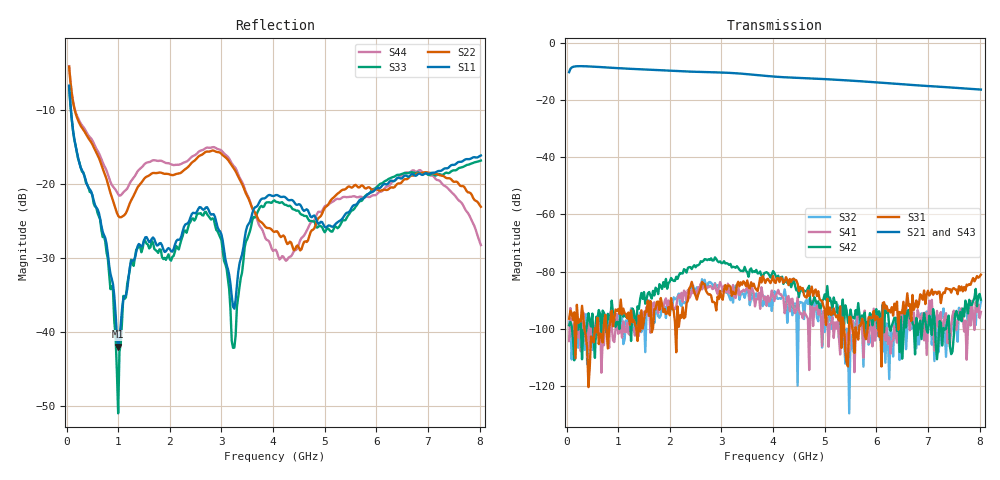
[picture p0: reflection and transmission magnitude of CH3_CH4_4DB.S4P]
!Agilent Technologies,E5071C,MY46316741,A.11.02
!Date: Thu May 28 15:03:34 2026
!Data & Calibration Information:
!1:CH3 INPUT 2:CH3 OUTPUT 3:CH4 INPUT 4:CH4 OUTPUT
!Freq	S11:SOLT4(ON)	S12:SOLT4(ON)	S13:SOLT4(ON)	S14:SOLT4(ON)
!	S21:SOLT4(ON)	S22:SOLT4(ON)	S23:SOLT4(ON)	S24:SOLT4(ON)
!	S31:SOLT4(ON)	S32:SOLT4(ON)	S33:SOLT4(ON)	S34:SOLT4(ON)
!	S41:SOLT4(ON)	S42:SOLT4(ON)	S43:SOLT4(ON)	S44:SOLT4(ON)
!PortZ  Port1:50+j0  Port2:50+j0  Port3:50+j0  Port4:50+j0
!Above PortZ is port z conversion or system Z0 setting when saving the data.
!When reading, reference impedance value at option line is always used.
# Hz S dB R 50
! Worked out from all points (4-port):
!   320 points, 50 MHz to 8.025 GHz, reference 50 ohm
!   strongest paths, dB at 50 MHz, 2.05 GHz, 4.05 GHz, 6.05 GHz, 8.025 GHz:
!     S21: -10.3, -9.8, -11.9, -13.9, -16.4
!     S43: -10.3, -9.9, -11.9, -14.0, -16.6
!     S31: -96.5, -93.0, -84.0, -102.7, -81.1
!     S42: -98.8, -82.9, -81.5, -93.9, -89.9
!     S41: -104.3, -91.3, -88.4, -99.8, -94.1
!     S32: -98.2, -91.9, -87.4, -101.2, -90.7
!   lowest |S11| = -42.0 dB at 1 GHz (marker M1), VSWR 1.02, Z = 49.3 - j0.315 ohm
!   |S11| at or under -10 dB: 85.51 MHz to end of sweep
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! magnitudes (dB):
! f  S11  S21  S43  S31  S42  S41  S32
! 50 MHz  -6.8  -10.3  -10.3  -96.5  -98.8  -104.3  -98.2
! 1 GHz  -42.0  -8.9  -8.9  -93.1  -97.6  -101.8  -97.6
! 1.5 GHz  -27.7  -9.4  -9.4  -97.0  -87.2  -94.0  -94.9
! 2.85 GHz  -24.1  -10.4  -10.4  -90.6  -76.1  -85.9  -85.6
! 3.25 GHz  -36.8  -10.7  -10.7  -87.8  -78.4  -88.9  -86.1
! 3.775 GHz  -22.0  -11.5  -11.5  -83.8  -81.5  -85.5  -90.5
! 8.025 GHz  -16.2  -16.4  -16.6  -81.1  -89.9  -94.1  -90.7
